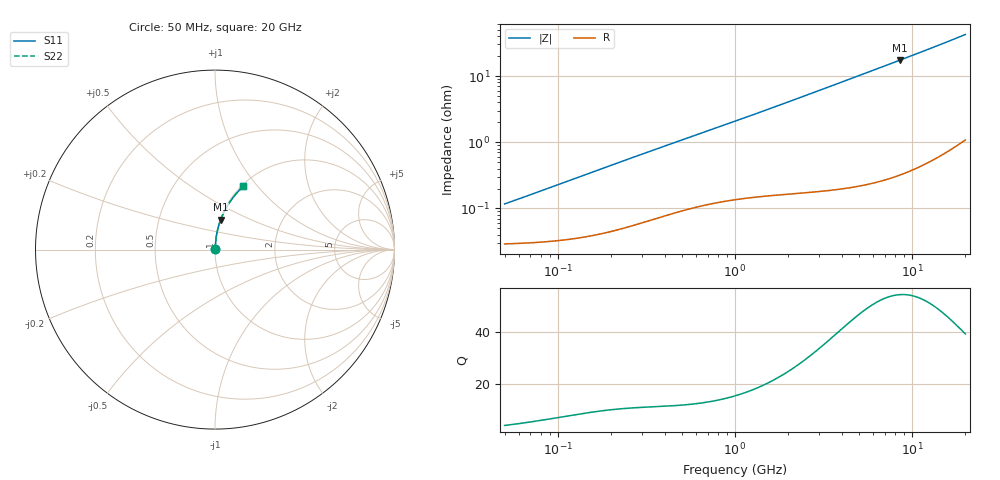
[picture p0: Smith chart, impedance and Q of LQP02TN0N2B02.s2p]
!Murata Part Number: LQP02TN0N2B02
!These Parameters are Measured in Series Mode Connection
!  o--[Z]--o
!Port1  Port2
!  o-------o
!Freq. Start=50[MHz] Stop=20[GHz], 401[Steps]
# Hz S RI R 50
!Freq.(Hz) S11(Real) S11(Imag) S21(Real) S21(Imag) S12(Real) S12(Imag) S22(Real) S22(Imag)
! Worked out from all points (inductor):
!   401 points, 50 MHz to 20 GHz, reference 50 ohm
!   read as one part in series: L = 360 pH near 51.52 MHz
!   highest Q = 54.3 at 8.516 GHz (marker M1), where L = 323 pH
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5e7  0.000293 0.00113  0.9997 -0.00113  0.9997 -0.00113  0.000293 0.00113
5.152053e7  0.000293 0.00117  0.9997 -0.00117  0.9997 -0.00117  0.000293 0.00117
6.354076e7  0.000301 0.00144  0.9997 -0.00144  0.9997 -0.00144  0.000301 0.00144
1.364002e8  0.000374 0.00307  0.9996 -0.00307  0.9996 -0.00307  0.000374 0.00307
2.33884e8  0.000528 0.0052  0.9995 -0.0052  0.9995 -0.0052  0.000528 0.0052
3.721004e8  0.000791 0.00811  0.9992 -0.00811  0.9992 -0.00811  0.000791 0.00811
6.380365e8  0.00126 0.0135  0.9987 -0.0135  0.9987 -0.0135  0.00126 0.0135
1e9  0.00178 0.0206  0.9982 -0.0206  0.9982 -0.0206  0.00178 0.0206
1.714689e9  0.0028 0.0348  0.9972 -0.0348  0.9972 -0.0348  0.0028 0.0348
2.728004e9  0.00478 0.0548  0.9952 -0.0548  0.9952 -0.0548  0.00478 0.0548
3.626126e9  0.00721 0.0726  0.9928 -0.0726  0.9928 -0.0726  0.00721 0.0726
4.677679e9  0.0109 0.0933  0.9891 -0.0933  0.9891 -0.0933  0.0109 0.0933
5.944466e9  0.0165 0.118  0.9835 -0.118  0.9835 -0.118  0.0165 0.118
7.442007e9  0.0249 0.1467  0.9751 -0.1467  0.9751 -0.1467  0.0249 0.1467
8.516016e9  0.032 0.1669  0.968 -0.1669  0.968 -0.1669  0.032 0.1669
1.098561e10  0.0516 0.212  0.9484 -0.212  0.9484 -0.212  0.0516 0.212
1.354865e10  0.0767 0.2562  0.9233 -0.2562  0.9233 -0.2562  0.0767 0.2562
1.482269e10  0.0908 0.277  0.9092 -0.277  0.9092 -0.277  0.0908 0.277
1.621653e10  0.1075 0.2989  0.8925 -0.2989  0.8925 -0.2989  0.1075 0.2989
1.774144e10  0.1271 0.3216  0.8729 -0.3216  0.8729 -0.3216  0.1271 0.3216
1.940974e10  0.15 0.3448  0.85 -0.3448  0.85 -0.3448  0.15 0.3448
2e10  0.1585 0.3527  0.8415 -0.3527  0.8415 -0.3527  0.1585 0.3527
